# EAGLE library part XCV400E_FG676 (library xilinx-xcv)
xcv400e_fg676 edit this description Auto generated by make-symbol-device-package-bsdl.ulp Rev. 26 Source: xcv400e_fg676.bsd
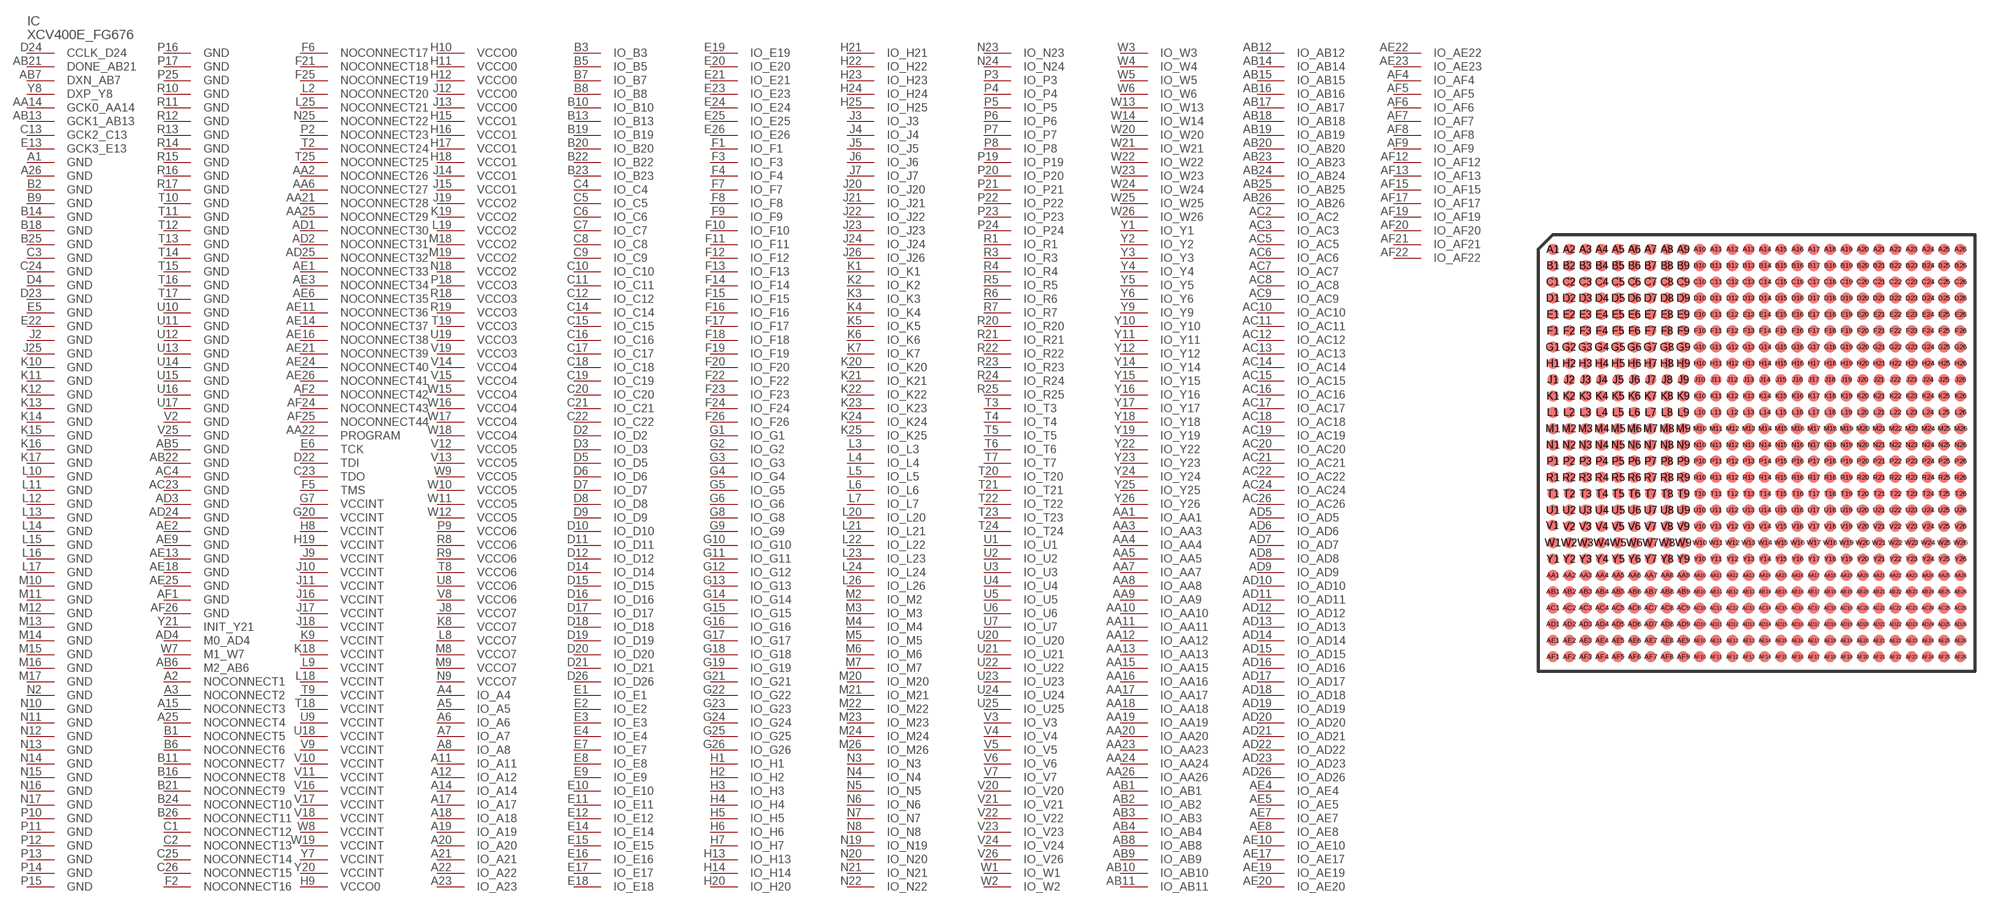
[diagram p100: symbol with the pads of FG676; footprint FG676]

Designator prefix IC

## XCV400E_FG676 (OC_FARNELL: unknown; OC_NEWARK: unknown)  [FG676]
A1  GND  pwr
A2  NOCONNECT1  pas
A3  NOCONNECT2  pas
A4  IO_A4
A5  IO_A5
A6  IO_A6
A7  IO_A7
A8  IO_A8
A11  IO_A11
A12  IO_A12
A14  IO_A14
A15  NOCONNECT3  pas
A17  IO_A17
A18  IO_A18
A19  IO_A19
A20  IO_A20
A21  IO_A21
A22  IO_A22
A23  IO_A23
A25  NOCONNECT4  pas
A26  GND  pwr
AA1  IO_AA1
AA2  NOCONNECT26  pas
AA3  IO_AA3
AA4  IO_AA4
AA5  IO_AA5
AA6  NOCONNECT27  pas
AA7  IO_AA7
AA8  IO_AA8
AA9  IO_AA9
AA10  IO_AA10
AA11  IO_AA11
AA12  IO_AA12
AA13  IO_AA13
AA14  GCK0_AA14  in
AA15  IO_AA15
AA16  IO_AA16
AA17  IO_AA17
AA18  IO_AA18
AA19  IO_AA19
AA20  IO_AA20
AA21  NOCONNECT28  pas
AA22  PROGRAM  in
AA23  IO_AA23
AA24  IO_AA24
AA25  NOCONNECT29  pas
AA26  IO_AA26
AB1  IO_AB1
AB2  IO_AB2
AB3  IO_AB3
AB4  IO_AB4
AB5  GND  pwr
AB6  M2_AB6  in
AB7  DXN_AB7  pas
AB8  IO_AB8
AB9  IO_AB9
AB10  IO_AB10
AB11  IO_AB11
AB12  IO_AB12
AB13  GCK1_AB13  in
AB14  IO_AB14
AB15  IO_AB15
AB16  IO_AB16
AB17  IO_AB17
AB18  IO_AB18
AB19  IO_AB19
AB20  IO_AB20
AB21  DONE_AB21
AB22  GND  pwr
AB23  IO_AB23
AB24  IO_AB24
AB25  IO_AB25
AB26  IO_AB26
AC2  IO_AC2
AC3  IO_AC3
AC4  GND  pwr
AC5  IO_AC5
AC6  IO_AC6
AC7  IO_AC7
AC8  IO_AC8
AC9  IO_AC9
AC10  IO_AC10
AC11  IO_AC11
AC12  IO_AC12
AC13  IO_AC13
AC14  IO_AC14
AC15  IO_AC15
AC16  IO_AC16
AC17  IO_AC17
AC18  IO_AC18
AC19  IO_AC19
AC20  IO_AC20
AC21  IO_AC21
AC22  IO_AC22
AC23  GND  pwr
AC24  IO_AC24
AC26  IO_AC26
AD1  NOCONNECT30  pas
AD2  NOCONNECT31  pas
AD3  GND  pwr
AD4  M0_AD4  in
AD5  IO_AD5
AD6  IO_AD6
AD7  IO_AD7
AD8  IO_AD8
AD9  IO_AD9
AD10  IO_AD10
AD11  IO_AD11
AD12  IO_AD12
AD13  IO_AD13
AD14  IO_AD14
AD15  IO_AD15
AD16  IO_AD16
AD17  IO_AD17
AD18  IO_AD18
AD19  IO_AD19
AD20  IO_AD20
AD21  IO_AD21
AD22  IO_AD22
AD23  IO_AD23
AD24  GND  pwr
AD25  NOCONNECT32  pas
AD26  IO_AD26
AE1  NOCONNECT33  pas
AE2  GND  pwr
AE3  NOCONNECT34  pas
AE4  IO_AE4
AE5  IO_AE5
AE6  NOCONNECT35  pas
AE7  IO_AE7
AE8  IO_AE8
AE9  GND  pwr
AE10  IO_AE10
AE11  NOCONNECT36  pas
AE13  GND  pwr
AE14  NOCONNECT37  pas
AE16  NOCONNECT38  pas
AE17  IO_AE17
AE18  GND  pwr
AE19  IO_AE19
AE20  IO_AE20
AE21  NOCONNECT39  pas
AE22  IO_AE22
AE23  IO_AE23
AE24  NOCONNECT40  pas
AE25  GND  pwr
AE26  NOCONNECT41  pas
AF1  GND  pwr
AF2  NOCONNECT42  pas
AF4  IO_AF4
AF5  IO_AF5
AF6  IO_AF6
AF7  IO_AF7
AF8  IO_AF8
AF9  IO_AF9
AF12  IO_AF12
AF13  IO_AF13
AF15  IO_AF15
AF17  IO_AF17
AF19  IO_AF19
AF20  IO_AF20
AF21  IO_AF21
AF22  IO_AF22
AF24  NOCONNECT43  pas
AF25  NOCONNECT44  pas
AF26  GND  pwr
B1  NOCONNECT5  pas
B2  GND  pwr
B3  IO_B3
B5  IO_B5
B6  NOCONNECT6  pas
B7  IO_B7
B8  IO_B8
B9  GND  pwr
B10  IO_B10
B11  NOCONNECT7  pas
B13  IO_B13
B14  GND  pwr
B16  NOCONNECT8  pas
B18  GND  pwr
B19  IO_B19
B20  IO_B20
B21  NOCONNECT9  pas
B22  IO_B22
B23  IO_B23
B24  NOCONNECT10  pas
B25  GND  pwr
B26  NOCONNECT11  pas
C1  NOCONNECT12  pas
C2  NOCONNECT13  pas
C3  GND  pwr
C4  IO_C4
C5  IO_C5
C6  IO_C6
C7  IO_C7
C8  IO_C8
C9  IO_C9
C10  IO_C10
C11  IO_C11
C12  IO_C12
C13  GCK2_C13  in
C14  IO_C14
C15  IO_C15
C16  IO_C16
C17  IO_C17
C18  IO_C18
C19  IO_C19
C20  IO_C20
C21  IO_C21
C22  IO_C22
C23  TDO  out
C24  GND  pwr
C25  NOCONNECT14  pas
C26  NOCONNECT15  pas
D2  IO_D2
D3  IO_D3
D4  GND  pwr
D5  IO_D5
D6  IO_D6
D7  IO_D7
D8  IO_D8
D9  IO_D9
D10  IO_D10
D11  IO_D11
D12  IO_D12
D14  IO_D14
D15  IO_D15
D16  IO_D16
D17  IO_D17
D18  IO_D18
D19  IO_D19
D20  IO_D20
D21  IO_D21
D22  TDI  in
D23  GND  pwr
D24  CCLK_D24
D26  IO_D26
E1  IO_E1
E2  IO_E2
E3  IO_E3
E4  IO_E4
E5  GND  pwr
E6  TCK  in
E7  IO_E7
E8  IO_E8
E9  IO_E9
E10  IO_E10
E11  IO_E11
E12  IO_E12
E13  GCK3_E13  in
E14  IO_E14
E15  IO_E15
E16  IO_E16
E17  IO_E17
E18  IO_E18
E19  IO_E19
E20  IO_E20
E21  IO_E21
E22  GND  pwr
E23  IO_E23
E24  IO_E24
E25  IO_E25
E26  IO_E26
F1  IO_F1
F2  NOCONNECT16  pas
F3  IO_F3
F4  IO_F4
F5  TMS  in
F6  NOCONNECT17  pas
F7  IO_F7
F8  IO_F8
F9  IO_F9
F10  IO_F10
F11  IO_F11
F12  IO_F12
F13  IO_F13
F14  IO_F14
F15  IO_F15
F16  IO_F16
F17  IO_F17
F18  IO_F18
F19  IO_F19
F20  IO_F20
F21  NOCONNECT18  pas
F22  IO_F22
F23  IO_F23
F24  IO_F24
F25  NOCONNECT19  pas
F26  IO_F26
G1  IO_G1
G2  IO_G2
G3  IO_G3
G4  IO_G4
G5  IO_G5
G6  IO_G6
G7  VCCINT  pwr
G8  IO_G8
G9  IO_G9
G10  IO_G10
G11  IO_G11
G12  IO_G12
G13  IO_G13
G14  IO_G14
G15  IO_G15
G16  IO_G16
G17  IO_G17
G18  IO_G18
G19  IO_G19
G20  VCCINT  pwr
G21  IO_G21
G22  IO_G22
G23  IO_G23
G24  IO_G24
G25  IO_G25
G26  IO_G26
H1  IO_H1
H2  IO_H2
H3  IO_H3
H4  IO_H4
H5  IO_H5
H6  IO_H6
H7  IO_H7
H8  VCCINT  pwr
H9  VCCO0  pwr
H10  VCCO0  pwr
H11  VCCO0  pwr
H12  VCCO0  pwr
H13  IO_H13
H14  IO_H14
H15  VCCO1  pwr
H16  VCCO1  pwr
H17  VCCO1  pwr
H18  VCCO1  pwr
H19  VCCINT  pwr
H20  IO_H20
H21  IO_H21
H22  IO_H22
H23  IO_H23
H24  IO_H24
H25  IO_H25
J2  GND  pwr
J3  IO_J3
J4  IO_J4
J5  IO_J5
J6  IO_J6
J7  IO_J7
J8  VCCO7  pwr
J9  VCCINT  pwr
J10  VCCINT  pwr
J11  VCCINT  pwr
J12  VCCO0  pwr
J13  VCCO0  pwr
J14  VCCO1  pwr
J15  VCCO1  pwr
J16  VCCINT  pwr
J17  VCCINT  pwr
J18  VCCINT  pwr
J19  VCCO2  pwr
J20  IO_J20
J21  IO_J21
J22  IO_J22
J23  IO_J23
J24  IO_J24
J25  GND  pwr
J26  IO_J26
K1  IO_K1
K2  IO_K2
K3  IO_K3
K4  IO_K4
K5  IO_K5
K6  IO_K6
K7  IO_K7
K8  VCCO7  pwr
K9  VCCINT  pwr
K10  GND  pwr
K11  GND  pwr
K12  GND  pwr
K13  GND  pwr
K14  GND  pwr
K15  GND  pwr
K16  GND  pwr
K17  GND  pwr
K18  VCCINT  pwr
K19  VCCO2  pwr
K20  IO_K20
K21  IO_K21
K22  IO_K22
K23  IO_K23
K24  IO_K24
K25  IO_K25
L2  NOCONNECT20  pas
L3  IO_L3
L4  IO_L4
L5  IO_L5
L6  IO_L6
L7  IO_L7
L8  VCCO7  pwr
L9  VCCINT  pwr
L10  GND  pwr
L11  GND  pwr
L12  GND  pwr
L13  GND  pwr
L14  GND  pwr
L15  GND  pwr
L16  GND  pwr
L17  GND  pwr
L18  VCCINT  pwr
L19  VCCO2  pwr
L20  IO_L20
L21  IO_L21
L22  IO_L22
L23  IO_L23
L24  IO_L24
L25  NOCONNECT21  pas
L26  IO_L26
M2  IO_M2
M3  IO_M3
M4  IO_M4
M5  IO_M5
M6  IO_M6
M7  IO_M7
M8  VCCO7  pwr
M9  VCCO7  pwr
M10  GND  pwr
M11  GND  pwr
M12  GND  pwr
M13  GND  pwr
M14  GND  pwr
M15  GND  pwr
M16  GND  pwr
M17  GND  pwr
M18  VCCO2  pwr
M19  VCCO2  pwr
M20  IO_M20
M21  IO_M21
M22  IO_M22
M23  IO_M23
M24  IO_M24
M26  IO_M26
N2  GND  pwr
N3  IO_N3
N4  IO_N4
N5  IO_N5
N6  IO_N6
N7  IO_N7
N8  IO_N8
N9  VCCO7  pwr
N10  GND  pwr
N11  GND  pwr
N12  GND  pwr
N13  GND  pwr
N14  GND  pwr
N15  GND  pwr
N16  GND  pwr
N17  GND  pwr
N18  VCCO2  pwr
N19  IO_N19
N20  IO_N20
N21  IO_N21
N22  IO_N22
N23  IO_N23
N24  IO_N24
N25  NOCONNECT22  pas
P2  NOCONNECT23  pas
P3  IO_P3
P4  IO_P4
P5  IO_P5
P6  IO_P6
P7  IO_P7
P8  IO_P8
P9  VCCO6  pwr
P10  GND  pwr
P11  GND  pwr
P12  GND  pwr
P13  GND  pwr
P14  GND  pwr
P15  GND  pwr
P16  GND  pwr
P17  GND  pwr
P18  VCCO3  pwr
P19  IO_P19
P20  IO_P20
P21  IO_P21
P22  IO_P22
P23  IO_P23
P24  IO_P24
P25  GND  pwr
R1  IO_R1
R3  IO_R3
R4  IO_R4
R5  IO_R5
R6  IO_R6
R7  IO_R7
R8  VCCO6  pwr
R9  VCCO6  pwr
R10  GND  pwr
R11  GND  pwr
R12  GND  pwr
R13  GND  pwr
R14  GND  pwr
R15  GND  pwr
R16  GND  pwr
R17  GND  pwr
R18  VCCO3  pwr
R19  VCCO3  pwr
R20  IO_R20
R21  IO_R21
R22  IO_R22
R23  IO_R23
R24  IO_R24
R25  IO_R25
T2  NOCONNECT24  pas
T3  IO_T3
T4  IO_T4
T5  IO_T5
T6  IO_T6
T7  IO_T7
T8  VCCO6  pwr
T9  VCCINT  pwr
T10  GND  pwr
T11  GND  pwr
T12  GND  pwr
T13  GND  pwr
T14  GND  pwr
T15  GND  pwr
T16  GND  pwr
T17  GND  pwr
T18  VCCINT  pwr
T19  VCCO3  pwr
T20  IO_T20
T21  IO_T21
T22  IO_T22
T23  IO_T23
T24  IO_T24
T25  NOCONNECT25  pas
U1  IO_U1
U2  IO_U2
U3  IO_U3
U4  IO_U4
U5  IO_U5
U6  IO_U6
U7  IO_U7
U8  VCCO6  pwr
U9  VCCINT  pwr
U10  GND  pwr
U11  GND  pwr
U12  GND  pwr
U13  GND  pwr
U14  GND  pwr
U15  GND  pwr
U16  GND  pwr
U17  GND  pwr
U18  VCCINT  pwr
U19  VCCO3  pwr
U20  IO_U20
U21  IO_U21
U22  IO_U22
U23  IO_U23
U24  IO_U24
U25  IO_U25
V2  GND  pwr
V3  IO_V3
V4  IO_V4
V5  IO_V5
V6  IO_V6
V7  IO_V7
V8  VCCO6  pwr
V9  VCCINT  pwr
V10  VCCINT  pwr
V11  VCCINT  pwr
V12  VCCO5  pwr
V13  VCCO5  pwr
V14  VCCO4  pwr
V15  VCCO4  pwr
V16  VCCINT  pwr
V17  VCCINT  pwr
V18  VCCINT  pwr
V19  VCCO3  pwr
V20  IO_V20
V21  IO_V21
V22  IO_V22
V23  IO_V23
V24  IO_V24
V25  GND  pwr
V26  IO_V26
W1  IO_W1
W2  IO_W2
W3  IO_W3
W4  IO_W4
W5  IO_W5
W6  IO_W6
W7  M1_W7  in
W8  VCCINT  pwr
W9  VCCO5  pwr
W10  VCCO5  pwr
W11  VCCO5  pwr
W12  VCCO5  pwr
W13  IO_W13
W14  IO_W14
W15  VCCO4  pwr
W16  VCCO4  pwr
W17  VCCO4  pwr
W18  VCCO4  pwr
W19  VCCINT  pwr
W20  IO_W20
W21  IO_W21
W22  IO_W22
W23  IO_W23
W24  IO_W24
W25  IO_W25
W26  IO_W26
Y1  IO_Y1
Y2  IO_Y2
Y3  IO_Y3
Y4  IO_Y4
Y5  IO_Y5
Y6  IO_Y6
Y7  VCCINT  pwr
Y8  DXP_Y8  pas
Y9  IO_Y9
Y10  IO_Y10
Y11  IO_Y11
Y12  IO_Y12
Y14  IO_Y14
Y15  IO_Y15
Y16  IO_Y16
Y17  IO_Y17
Y18  IO_Y18
Y19  IO_Y19
Y20  VCCINT  pwr
Y21  INIT_Y21
Y22  IO_Y22
Y23  IO_Y23
Y24  IO_Y24
Y25  IO_Y25
Y26  IO_Y26

## Footprint FG676 (pad centres in mm)
xcv400_fg676 edit this description Auto generated by make-symbol-device-package-bsdl.ulp Rev. 26 Source: xcv400_fg676.bsd
smd 0.7 x 0.7: A1 -12.5,12.5; A2 -11.5,12.5; A3 -10.5,12.5; A4 -9.5,12.5; A5 -8.5,12.5; A6 -7.5,12.5; A7 -6.5,12.5; A8 -5.5,12.5; A9 -4.5,12.5; A10 -3.5,12.5; A11 -2.5,12.5; A12 -1.5,12.5; A13 -0.5,12.5; A14 0.5,12.5; A15 1.5,12.5; A16 2.5,12.5; A17 3.5,12.5; A18 4.5,12.5; A19 5.5,12.5; A20 6.5,12.5; A21 7.5,12.5; A22 8.5,12.5; A23 9.5,12.5; A24 10.5,12.5; A25 11.5,12.5; A26 12.5,12.5; AA1 -12.5,-7.5; AA2 -11.5,-7.5; AA3 -10.5,-7.5; AA4 -9.5,-7.5; AA5 -8.5,-7.5; AA6 -7.5,-7.5; AA7 -6.5,-7.5; AA8 -5.5,-7.5; AA9 -4.5,-7.5; AA10 -3.5,-7.5; AA11 -2.5,-7.5; AA12 -1.5,-7.5; AA13 -0.5,-7.5; AA14 0.5,-7.5; AA15 1.5,-7.5; AA16 2.5,-7.5; AA17 3.5,-7.5; AA18 4.5,-7.5; AA19 5.5,-7.5; AA20 6.5,-7.5; AA21 7.5,-7.5; AA22 8.5,-7.5; AA23 9.5,-7.5; AA24 10.5,-7.5; AA25 11.5,-7.5; AA26 12.5,-7.5; AB1 -12.5,-8.5; AB2 -11.5,-8.5; AB3 -10.5,-8.5; AB4 -9.5,-8.5; AB5 -8.5,-8.5; AB6 -7.5,-8.5; AB7 -6.5,-8.5; AB8 -5.5,-8.5; AB9 -4.5,-8.5; AB10 -3.5,-8.5; AB11 -2.5,-8.5; AB12 -1.5,-8.5; AB13 -0.5,-8.5; AB14 0.5,-8.5; AB15 1.5,-8.5; AB16 2.5,-8.5; AB17 3.5,-8.5; AB18 4.5,-8.5; AB19 5.5,-8.5; AB20 6.5,-8.5; AB21 7.5,-8.5; AB22 8.5,-8.5; AB23 9.5,-8.5; AB24 10.5,-8.5; AB25 11.5,-8.5; AB26 12.5,-8.5; AC1 -12.5,-9.5; AC2 -11.5,-9.5; AC3 -10.5,-9.5; AC4 -9.5,-9.5; AC5 -8.5,-9.5; AC6 -7.5,-9.5; AC7 -6.5,-9.5; AC8 -5.5,-9.5; AC9 -4.5,-9.5; AC10 -3.5,-9.5; AC11 -2.5,-9.5; AC12 -1.5,-9.5; AC13 -0.5,-9.5; AC14 0.5,-9.5; AC15 1.5,-9.5; AC16 2.5,-9.5; AC17 3.5,-9.5; AC18 4.5,-9.5; AC19 5.5,-9.5; AC20 6.5,-9.5; AC21 7.5,-9.5; AC22 8.5,-9.5; AC23 9.5,-9.5; AC24 10.5,-9.5; AC25 11.5,-9.5; AC26 12.5,-9.5; AD1 -12.5,-10.5; AD2 -11.5,-10.5; AD3 -10.5,-10.5; AD4 -9.5,-10.5; AD5 -8.5,-10.5; AD6 -7.5,-10.5; AD7 -6.5,-10.5; AD8 -5.5,-10.5; AD9 -4.5,-10.5; AD10 -3.5,-10.5; AD11 -2.5,-10.5; AD12 -1.5,-10.5; AD13 -0.5,-10.5; AD14 0.5,-10.5; AD15 1.5,-10.5; AD16 2.5,-10.5; AD17 3.5,-10.5; AD18 4.5,-10.5; AD19 5.5,-10.5; AD20 6.5,-10.5; AD21 7.5,-10.5; AD22 8.5,-10.5; AD23 9.5,-10.5; AD24 10.5,-10.5; AD25 11.5,-10.5; AD26 12.5,-10.5; AE1 -12.5,-11.5; AE2 -11.5,-11.5; AE3 -10.5,-11.5; AE4 -9.5,-11.5; AE5 -8.5,-11.5; AE6 -7.5,-11.5; AE7 -6.5,-11.5; AE8 -5.5,-11.5; AE9 -4.5,-11.5; AE10 -3.5,-11.5; AE11 -2.5,-11.5; AE12 -1.5,-11.5; AE13 -0.5,-11.5; AE14 0.5,-11.5; AE15 1.5,-11.5; AE16 2.5,-11.5; AE17 3.5,-11.5; AE18 4.5,-11.5; AE19 5.5,-11.5; AE20 6.5,-11.5; AE21 7.5,-11.5; AE22 8.5,-11.5; AE23 9.5,-11.5; AE24 10.5,-11.5; AE25 11.5,-11.5; AE26 12.5,-11.5; AF1 -12.5,-12.5; AF2 -11.5,-12.5; AF3 -10.5,-12.5; AF4 -9.5,-12.5; AF5 -8.5,-12.5; AF6 -7.5,-12.5; AF7 -6.5,-12.5; AF8 -5.5,-12.5; AF9 -4.5,-12.5; AF10 -3.5,-12.5; AF11 -2.5,-12.5; AF12 -1.5,-12.5; AF13 -0.5,-12.5; AF14 0.5,-12.5; AF15 1.5,-12.5; AF16 2.5,-12.5; AF17 3.5,-12.5; AF18 4.5,-12.5; AF19 5.5,-12.5; AF20 6.5,-12.5; AF21 7.5,-12.5; AF22 8.5,-12.5; AF23 9.5,-12.5; AF24 10.5,-12.5; AF25 11.5,-12.5; AF26 12.5,-12.5; B1 -12.5,11.5; B2 -11.5,11.5; B3 -10.5,11.5; B4 -9.5,11.5; B5 -8.5,11.5; B6 -7.5,11.5; B7 -6.5,11.5; B8 -5.5,11.5; B9 -4.5,11.5; B10 -3.5,11.5; B11 -2.5,11.5; B12 -1.5,11.5; B13 -0.5,11.5; B14 0.5,11.5; B15 1.5,11.5; B16 2.5,11.5; B17 3.5,11.5; B18 4.5,11.5; B19 5.5,11.5; B20 6.5,11.5; B21 7.5,11.5; B22 8.5,11.5; B23 9.5,11.5; B24 10.5,11.5; B25 11.5,11.5; B26 12.5,11.5; C1 -12.5,10.5; C2 -11.5,10.5; C3 -10.5,10.5; C4 -9.5,10.5; C5 -8.5,10.5; C6 -7.5,10.5; C7 -6.5,10.5; C8 -5.5,10.5; C9 -4.5,10.5; C10 -3.5,10.5; C11 -2.5,10.5; C12 -1.5,10.5; C13 -0.5,10.5; C14 0.5,10.5; C15 1.5,10.5; C16 2.5,10.5; C17 3.5,10.5; C18 4.5,10.5; C19 5.5,10.5; C20 6.5,10.5; C21 7.5,10.5; C22 8.5,10.5; C23 9.5,10.5; C24 10.5,10.5; C25 11.5,10.5; C26 12.5,10.5; D1 -12.5,9.5; D2 -11.5,9.5; D3 -10.5,9.5; D4 -9.5,9.5; D5 -8.5,9.5; D6 -7.5,9.5; D7 -6.5,9.5; D8 -5.5,9.5; D9 -4.5,9.5; D10 -3.5,9.5; D11 -2.5,9.5; D12 -1.5,9.5; D13 -0.5,9.5; D14 0.5,9.5; D15 1.5,9.5; D16 2.5,9.5; D17 3.5,9.5; D18 4.5,9.5; D19 5.5,9.5; D20 6.5,9.5; D21 7.5,9.5; D22 8.5,9.5; D23 9.5,9.5; D24 10.5,9.5; D25 11.5,9.5; D26 12.5,9.5; E1 -12.5,8.5; E2 -11.5,8.5; E3 -10.5,8.5; E4 -9.5,8.5; E5 -8.5,8.5; E6 -7.5,8.5; E7 -6.5,8.5; E8 -5.5,8.5; E9 -4.5,8.5; E10 -3.5,8.5; E11 -2.5,8.5; E12 -1.5,8.5; E13 -0.5,8.5; E14 0.5,8.5; E15 1.5,8.5; E16 2.5,8.5; E17 3.5,8.5; E18 4.5,8.5; E19 5.5,8.5; E20 6.5,8.5; E21 7.5,8.5; E22 8.5,8.5; E23 9.5,8.5; E24 10.5,8.5; E25 11.5,8.5; E26 12.5,8.5; F1 -12.5,7.5; F2 -11.5,7.5; F3 -10.5,7.5; F4 -9.5,7.5; F5 -8.5,7.5; F6 -7.5,7.5; F7 -6.5,7.5; F8 -5.5,7.5; F9 -4.5,7.5; F10 -3.5,7.5; F11 -2.5,7.5; F12 -1.5,7.5; F13 -0.5,7.5; F14 0.5,7.5; F15 1.5,7.5; F16 2.5,7.5; F17 3.5,7.5; F18 4.5,7.5; F19 5.5,7.5; F20 6.5,7.5; F21 7.5,7.5; F22 8.5,7.5; F23 9.5,7.5; F24 10.5,7.5; F25 11.5,7.5; F26 12.5,7.5; G1 -12.5,6.5; G2 -11.5,6.5; G3 -10.5,6.5; G4 -9.5,6.5; G5 -8.5,6.5; G6 -7.5,6.5; G7 -6.5,6.5; G8 -5.5,6.5; G9 -4.5,6.5; G10 -3.5,6.5; G11 -2.5,6.5; G12 -1.5,6.5; G13 -0.5,6.5; G14 0.5,6.5; G15 1.5,6.5; G16 2.5,6.5; G17 3.5,6.5; G18 4.5,6.5; G19 5.5,6.5; G20 6.5,6.5; G21 7.5,6.5; G22 8.5,6.5; G23 9.5,6.5; G24 10.5,6.5; G25 11.5,6.5; G26 12.5,6.5; H1 -12.5,5.5; H2 -11.5,5.5; H3 -10.5,5.5; H4 -9.5,5.5; H5 -8.5,5.5; H6 -7.5,5.5; H7 -6.5,5.5; H8 -5.5,5.5; H9 -4.5,5.5; H10 -3.5,5.5; H11 -2.5,5.5; H12 -1.5,5.5; H13 -0.5,5.5; H14 0.5,5.5; H15 1.5,5.5; H16 2.5,5.5; H17 3.5,5.5; H18 4.5,5.5; H19 5.5,5.5; H20 6.5,5.5; H21 7.5,5.5; H22 8.5,5.5; H23 9.5,5.5; H24 10.5,5.5; H25 11.5,5.5; H26 12.5,5.5; J1 -12.5,4.5; J2 -11.5,4.5; J3 -10.5,4.5; J4 -9.5,4.5; J5 -8.5,4.5; J6 -7.5,4.5; J7 -6.5,4.5; J8 -5.5,4.5; J9 -4.5,4.5; J10 -3.5,4.5; J11 -2.5,4.5; J12 -1.5,4.5; J13 -0.5,4.5; J14 0.5,4.5; J15 1.5,4.5; J16 2.5,4.5; J17 3.5,4.5; J18 4.5,4.5; J19 5.5,4.5; J20 6.5,4.5; J21 7.5,4.5; J22 8.5,4.5; J23 9.5,4.5; J24 10.5,4.5; J25 11.5,4.5; J26 12.5,4.5; K1 -12.5,3.5; K2 -11.5,3.5; K3 -10.5,3.5; K4 -9.5,3.5; K5 -8.5,3.5; K6 -7.5,3.5; K7 -6.5,3.5; K8 -5.5,3.5; K9 -4.5,3.5; K10 -3.5,3.5; K11 -2.5,3.5; K12 -1.5,3.5; K13 -0.5,3.5; K14 0.5,3.5; K15 1.5,3.5; K16 2.5,3.5; K17 3.5,3.5; K18 4.5,3.5; K19 5.5,3.5; K20 6.5,3.5; K21 7.5,3.5; K22 8.5,3.5; K23 9.5,3.5; K24 10.5,3.5; K25 11.5,3.5; K26 12.5,3.5; L1 -12.5,2.5; L2 -11.5,2.5; L3 -10.5,2.5; L4 -9.5,2.5; L5 -8.5,2.5; L6 -7.5,2.5; L7 -6.5,2.5; L8 -5.5,2.5; L9 -4.5,2.5; L10 -3.5,2.5; L11 -2.5,2.5; L12 -1.5,2.5; L13 -0.5,2.5; L14 0.5,2.5; L15 1.5,2.5; L16 2.5,2.5; L17 3.5,2.5; L18 4.5,2.5; L19 5.5,2.5; L20 6.5,2.5; L21 7.5,2.5; L22 8.5,2.5; L23 9.5,2.5; L24 10.5,2.5; L25 11.5,2.5; L26 12.5,2.5; M1 -12.5,1.5; M2 -11.5,1.5; M3 -10.5,1.5; M4 -9.5,1.5; M5 -8.5,1.5; M6 -7.5,1.5; M7 -6.5,1.5; M8 -5.5,1.5; M9 -4.5,1.5; M10 -3.5,1.5; M11 -2.5,1.5; M12 -1.5,1.5; M13 -0.5,1.5; M14 0.5,1.5; M15 1.5,1.5; M16 2.5,1.5; M17 3.5,1.5; M18 4.5,1.5; M19 5.5,1.5; M20 6.5,1.5; M21 7.5,1.5; M22 8.5,1.5; M23 9.5,1.5; M24 10.5,1.5; M25 11.5,1.5; M26 12.5,1.5; N1 -12.5,0.5; N2 -11.5,0.5; N3 -10.5,0.5; N4 -9.5,0.5; N5 -8.5,0.5; N6 -7.5,0.5; N7 -6.5,0.5; N8 -5.5,0.5; N9 -4.5,0.5; N10 -3.5,0.5; N11 -2.5,0.5; N12 -1.5,0.5; N13 -0.5,0.5; N14 0.5,0.5; N15 1.5,0.5; N16 2.5,0.5; N17 3.5,0.5; N18 4.5,0.5; N19 5.5,0.5; N20 6.5,0.5; N21 7.5,0.5; N22 8.5,0.5; N23 9.5,0.5; N24 10.5,0.5; N25 11.5,0.5; N26 12.5,0.5; P1 -12.5,-0.5; P2 -11.5,-0.5; P3 -10.5,-0.5; P4 -9.5,-0.5; P5 -8.5,-0.5; P6 -7.5,-0.5; P7 -6.5,-0.5; P8 -5.5,-0.5; P9 -4.5,-0.5; P10 -3.5,-0.5; P11 -2.5,-0.5; P12 -1.5,-0.5; P13 -0.5,-0.5; P14 0.5,-0.5; P15 1.5,-0.5; P16 2.5,-0.5; P17 3.5,-0.5; P18 4.5,-0.5; P19 5.5,-0.5; P20 6.5,-0.5; P21 7.5,-0.5; P22 8.5,-0.5; P23 9.5,-0.5; P24 10.5,-0.5; P25 11.5,-0.5; P26 12.5,-0.5; R1 -12.5,-1.5; R2 -11.5,-1.5; R3 -10.5,-1.5; R4 -9.5,-1.5; R5 -8.5,-1.5; R6 -7.5,-1.5; R7 -6.5,-1.5; R8 -5.5,-1.5; R9 -4.5,-1.5; R10 -3.5,-1.5; R11 -2.5,-1.5; R12 -1.5,-1.5; R13 -0.5,-1.5; R14 0.5,-1.5; R15 1.5,-1.5; R16 2.5,-1.5; R17 3.5,-1.5; R18 4.5,-1.5; R19 5.5,-1.5; R20 6.5,-1.5; R21 7.5,-1.5; R22 8.5,-1.5; R23 9.5,-1.5; R24 10.5,-1.5; R25 11.5,-1.5; R26 12.5,-1.5; T1 -12.5,-2.5; T2 -11.5,-2.5; T3 -10.5,-2.5; T4 -9.5,-2.5; T5 -8.5,-2.5; T6 -7.5,-2.5; T7 -6.5,-2.5; T8 -5.5,-2.5; T9 -4.5,-2.5; T10 -3.5,-2.5; T11 -2.5,-2.5; T12 -1.5,-2.5; T13 -0.5,-2.5; T14 0.5,-2.5; T15 1.5,-2.5; T16 2.5,-2.5; T17 3.5,-2.5; T18 4.5,-2.5; T19 5.5,-2.5; T20 6.5,-2.5; T21 7.5,-2.5; T22 8.5,-2.5; T23 9.5,-2.5; T24 10.5,-2.5; T25 11.5,-2.5; T26 12.5,-2.5; U1 -12.5,-3.5; U2 -11.5,-3.5; U3 -10.5,-3.5; U4 -9.5,-3.5; U5 -8.5,-3.5; U6 -7.5,-3.5; U7 -6.5,-3.5; U8 -5.5,-3.5; U9 -4.5,-3.5; U10 -3.5,-3.5; U11 -2.5,-3.5; U12 -1.5,-3.5; U13 -0.5,-3.5; U14 0.5,-3.5; U15 1.5,-3.5; U16 2.5,-3.5; U17 3.5,-3.5; U18 4.5,-3.5; U19 5.5,-3.5; U20 6.5,-3.5; U21 7.5,-3.5; U22 8.5,-3.5; U23 9.5,-3.5; U24 10.5,-3.5; U25 11.5,-3.5; U26 12.5,-3.5; V1 -12.527,-4.431; V2 -11.5,-4.5; V3 -10.5,-4.5; V4 -9.5,-4.5; V5 -8.5,-4.5; V6 -7.5,-4.5; V7 -6.5,-4.5; V8 -5.5,-4.5; V9 -4.5,-4.5; V10 -3.5,-4.5; V11 -2.5,-4.5; V12 -1.5,-4.5; V13 -0.5,-4.5; V14 0.5,-4.5; V15 1.5,-4.5; V16 2.5,-4.5; V17 3.5,-4.5; V18 4.5,-4.5; V19 5.5,-4.5; V20 6.5,-4.5; V21 7.5,-4.5; V22 8.5,-4.5; V23 9.5,-4.5; V24 10.5,-4.5; V25 11.5,-4.5; V26 12.5,-4.5; W1 -12.5,-5.5; W2 -11.5,-5.5; W3 -10.5,-5.5; W4 -9.5,-5.5; W5 -8.5,-5.5; W6 -7.5,-5.5; W7 -6.5,-5.5; W8 -5.5,-5.5; W9 -4.5,-5.5; W10 -3.5,-5.5; W11 -2.5,-5.5; W12 -1.5,-5.5; W13 -0.5,-5.5; W14 0.5,-5.5; W15 1.5,-5.5; W16 2.5,-5.5; W17 3.5,-5.5; W18 4.5,-5.5; W19 5.5,-5.5; W20 6.5,-5.5; W21 7.5,-5.5; W22 8.5,-5.5; W23 9.5,-5.5; W24 10.5,-5.5; W25 11.5,-5.5; W26 12.5,-5.5; Y1 -12.5,-6.5; Y2 -11.5,-6.5; Y3 -10.5,-6.5; Y4 -9.5,-6.5; Y5 -8.5,-6.5; Y6 -7.5,-6.5; Y7 -6.5,-6.5; Y8 -5.5,-6.5; Y9 -4.5,-6.5; Y10 -3.5,-6.5; Y11 -2.5,-6.5; Y12 -1.5,-6.5; Y13 -0.5,-6.5; Y14 0.5,-6.5; Y15 1.5,-6.5; Y16 2.5,-6.5; Y17 3.5,-6.5; Y18 4.5,-6.5; Y19 5.5,-6.5; Y20 6.5,-6.5; Y21 7.5,-6.5; Y22 8.5,-6.5; Y23 9.5,-6.5; Y24 10.5,-6.5; Y25 11.5,-6.5; Y26 12.5,-6.5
